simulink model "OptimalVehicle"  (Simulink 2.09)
settings: Solver=ode45  StartTime=0.0  StopTime=25  MaxStep=10  RelTol=1e-3  AbsTol=1e-3
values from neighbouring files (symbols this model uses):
  k = (1/ks)*(sqrt(1+(q/r)*ks^2)-1)    [VdataC.m]
  ki = 0.1    [VdataC.m]
  ks = ktheta/kv    [VdataC.m]
  T = 2.5    [HdataF.m]    (also in Mdata.m = 0.5; Mdata25.m = 0.5; VdataC.m = 0.25; VdataF.m = 0.25)
  theta0 = ((1/gamma)*(alpha*v0^2-Fi))^2    (= 0.186624)    [VdataM.m]
  v0 = 40    [VdataM.m]
  vd = 45    [VdataM.m]
undefined symbols (not defined in the file or in its folder): sfunyst
libraries: fuzzy x1

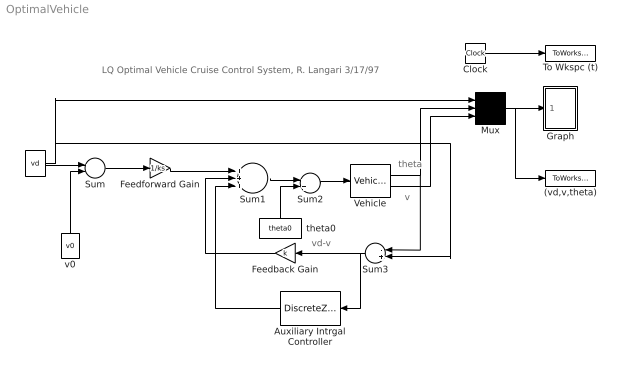
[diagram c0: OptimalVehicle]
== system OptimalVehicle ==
  note: v
  note: theta
  note: LQ Optimal Vehicle Cruise Control System, R. Langari 3/17/97
  note: vd-v
  " " : Constant  Value=vd
  (vd,v,theta) : ToWorkspace  VariableName=yout  SampleTime=0
  Auxiliary Intrgal Controller : DiscreteZeroPole  Orientation=left  Zeros=[]  Poles=[1]  Gain=[ki]  SampleTime=T
  Clock : Clock
  Feedback Gain : Gain  Orientation=left  Gain=k
  Feedforward Gain : Gain  Gain=1/ks
  Graph : Subsystem  mask(Storage scope.){}
      mask help: Storage scope using MATLAB graph window. Enter plotting ranges and line type.
      mask init:
      | npts = @4; color = @5; ax = [0, @1, @2, @3]; dt=-1;
  Mux : Mux  Inputs=3
  Sum : Sum  Inputs=+-
  Sum1 : Sum  Inputs=+++
  Sum2 : Sum  Inputs=++
  Sum3 : Sum  Orientation=left  Inputs=-+
  To Wkspc (t) : ToWorkspace  VariableName=t  SampleTime=0
  Vehicle : fuzzy/Vehicle
  theta0 : Constant  Orientation=up  Value=theta0
  v0 : Constant  Orientation=up  Value=v0
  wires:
  Vehicle/2 -> Mux/3
  Sum2/1 -> Vehicle/1
  Sum3/1 -> Auxiliary Intrgal Controller/1, Feedback Gain/1
  Auxiliary Intrgal Controller/1 -> Sum1/3
  Clock/1 -> To Wkspc (t)/1
  Mux/1 -> (vd,v,theta)/1, Graph/1(x)
  " "/1 -> Mux/1, Sum3/2, Sum/1
  theta0/1 -> Sum2/2
  Sum1/1 -> Sum2/1
  Feedback Gain/1 -> Sum1/2
  Feedforward Gain/1 -> Sum1/1
  Sum/1 -> Feedforward Gain/1
  v0/1 -> Sum/2
  Vehicle/1 -> Sum3/1, Mux/2

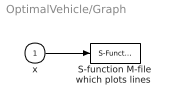
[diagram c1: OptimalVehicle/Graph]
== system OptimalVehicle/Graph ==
  x : Inport  Port=1  PortWidth=-1  SampleTime=-1
  "S-function M-file which plots lines " : S-Function  LoadFcn=sfunyst([],[],[],'LoadBlock')  FunctionName=sfunyst  Parameters=ax, color, npts, dt
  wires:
  x/1 -> "S-function M-file which plots lines "/1
